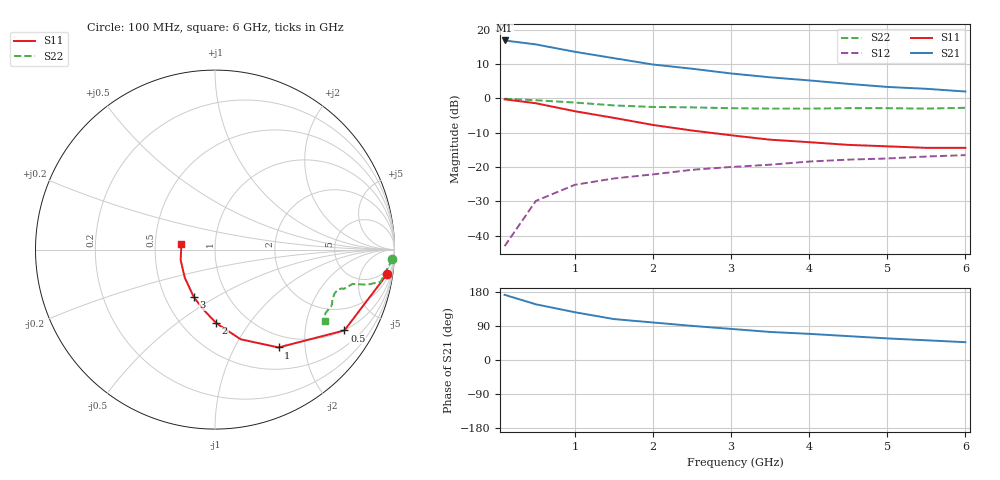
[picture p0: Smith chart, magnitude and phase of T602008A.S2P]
!AT-60200
!S-PARAMETERS at Vce=8V  Ic=1mA.  LAST UPDATED 07-21-92
# ghz s ma r 50
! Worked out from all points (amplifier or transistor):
!   13 points, 100 MHz to 6 GHz, reference 50 ohm
!   highest |S21| = 16.9 dB at 100 MHz (marker M1)
!   |S21| within 3 dB of that: start of sweep to 927.5 MHz
!   unconditionally stable (mu >= 1): 2.76 GHz to end of sweep
!   at 1 GHz: K = 0.50, MSG = 19.4 dB, |S12| = -25.2 dB
!   at 3 GHz: K = 1.05, MAG = 12.2 dB, |S12| = -20.0 dB
!   at 6 GHz: K = 1.17, MAG = 6.8 dB, |S12| = -16.5 dB
!   S11 on the Smith chart (normalised r, x): 100 MHz: 3, -14; 500 MHz: 0.99, -3.21; 1 GHz: 0.81, -1.53; 2 GHz: 0.72, -0.71; 3 GHz: 0.69, -0.40; 6 GHz: 0.68, +0.04
0.1  0.97 -8.0  7 172.0  0.007 87.0  0.99 -3.0
0.5  0.85 -32.0  6.13 147.0  0.032 73.0  0.94 -11.0
1  0.65 -57.0  4.78 126.0  0.055 64.0  0.87 -13.0
1.5  0.52 -74.0  3.86 108.0  0.068 59.0  0.79 -14.0
2  0.41 -89.0  3.12 99.0  0.078 58.0  0.75 -17.0
2.5  0.34 -101.0  2.71 90.0  0.091 59.0  0.74 -17.0
3  0.29 -114.0  2.31 82.0  0.1 61.0  0.72 -18.0
3.5  0.25 -126.0  2.03 74.0  0.108 60.0  0.71 -20.0
4  0.23 -137.0  1.83 69.0  0.12 61.0  0.71 -23.0
4.5  0.21 -149.0  1.63 63.0  0.128 60.0  0.72 -25.0
5  0.2 -163.0  1.47 57.0  0.133 61.0  0.72 -26.0
5.5  0.19 -175.0  1.38 52.0  0.142 61.0  0.71 -30.0
6  0.19 171.0  1.26 47.0  0.149 61.0  0.73 -33.0
